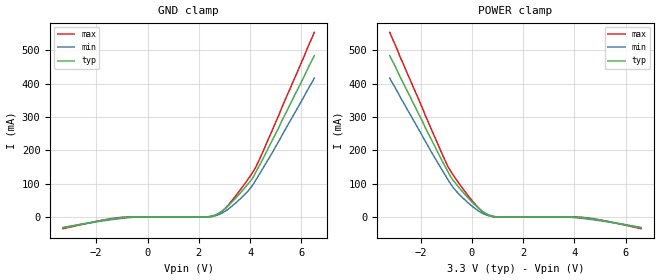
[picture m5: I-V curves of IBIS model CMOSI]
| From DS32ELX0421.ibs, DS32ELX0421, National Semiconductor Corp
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|   Model CMOSI
[Model]  CMOSI
Model_type Input
Vinl =   0
Vinh =   2
C_comp   914fF   914fF   914fF
[Temperature Range]   25.0000   85.0000   -40.0000
[Voltage Range]   3.3000V   3.0000V   3.4650V
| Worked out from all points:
|   GND clamp passes 1 mA (typ) near -0.90 V on its own axis
[GND_clamp]
|Voltage   I(typ)   I(min)   I(max)
-3.3V     -31.9mA    -31.3mA    -34.7mA
-1.12V    -2.7mA     -4.88mA    -1.53mA
-429mV    -628nA     -191uA     -1nA
2.24V     455uA      327uA      117uA
2.54V     3.84mA     2.42mA     2.3mA
2.84V     14.8mA     9.63mA     13.5mA
3.14V     33.4mA     23.5mA     35.4mA
3.63V     73.4mA     56mA       83.1mA
4.03V     110mA      88.5mA     126mA
4.22V     135mA      111mA      150mA
4.92V     239mA      201mA      271mA
6.5V      484mA      417mA      554mA
|6.60E+00   5.00E-01   4.31E-01   5.71E-01
[POWER_clamp]
|Voltage   I(typ)   I(min)   I(max)
-3.2V     484mA      417mA      554mA
-1.62V    239mA      201mA      271mA
-924mV    135mA      111mA      150mA
-726mV    110mA      88.5mA     126mA
-330mV    73.4mA     56mA       83.1mA
165mV     33.4mA     23.5mA     35.4mA
462mV     14.8mA     9.63mA     13.5mA
759mV     3.84mA     2.42mA     2.3mA
1.06V     455uA      327uA      117uA
3.73V     -628nA     -191uA     -1nA
4.42V     -2.7mA     -4.88mA    -1.53mA
6.6V      -31.9mA    -31.3mA    -34.7mA
